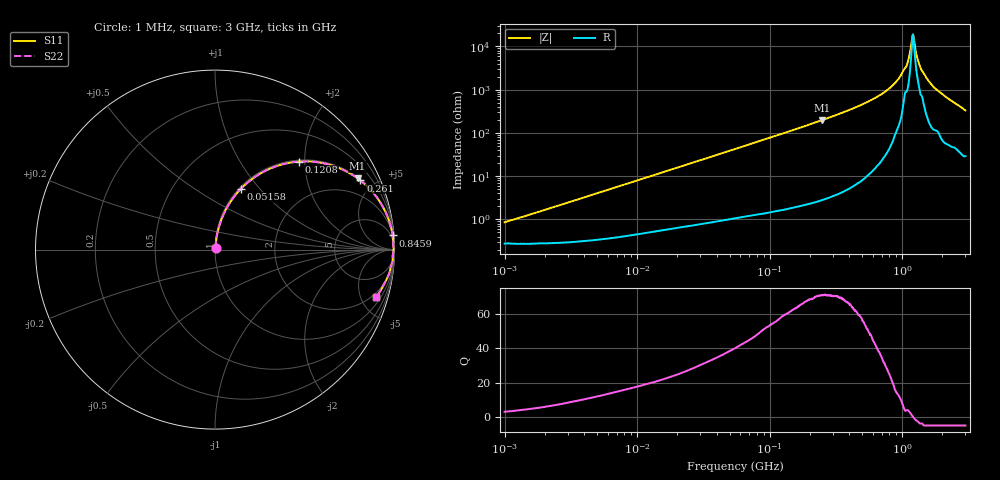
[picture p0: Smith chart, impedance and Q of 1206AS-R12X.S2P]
!s-Parameter Generated by FASTRON Sdn. Bhd.
!FASTRON P/N : 1206AS-R12X
!Keysight Technologies: E4991B_MY54100416_A.01.15
!Date: Wed Nov 15 11:00:45 2023
!Version  :Rev00  Wed Nov 15 11:00:45 2023
!Data & Calibration Information:
!Freq  S11  S21  S12  S22
!PortZ  Port1:50+j0  Port2:50+j0
!When reading reference impedance value at option line is always used.
! Remarks : This data is being provided solely for informational purposes.
# Hz S dB R 50
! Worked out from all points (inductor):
!   1601 points, 1 MHz to 3 GHz, reference 50 ohm
!   read as one part in series: L = 130 nH near 1.041 MHz
!   highest Q = 71 at 249.5 MHz (marker M1), where L = 127 nH
!   self-resonance near 1.207 GHz
!   S11 on the Smith chart (normalised r, x): 1 MHz: 1.01, +0.02; 51.58 MHz: 1.02, +0.80; 120.8 MHz: 1.03, +1.87; 261 MHz: 1.06, +4.17; 845.9 MHz: 2, +25; 3 GHz: 1.58, -6.61
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1000000  -41.33 70.8  -0.02 -0.5  -0.02 -0.5  -41.33 70.8
3804036  -30.23 82.5  -0.03 -1.8  -0.03 -1.8  -30.23 82.5
1.447069e7  -18.94 80.8  -0.10 -6.5  -0.10 -6.5  -18.94 80.8
5.15801e7  -8.69 67.0  -0.72 -21.6  -0.72 -21.6  -8.69 67.0
5.477226e7  -8.25 65.8  -0.80 -22.8  -0.80 -22.8  -8.25 65.8
1.207609e8  -3.39 46.4  -2.80 -42.6  -2.80 -42.6  -3.39 46.4
2.083556e8  -1.43 31.2  -5.72 -58.0  -5.72 -58.0  -1.43 31.2
2.494827e8  -1.03 26.6  -6.99 -62.6  -6.99 -62.6  -1.03 26.6
2.609752e8  -0.95 25.5  -7.33 -63.7  -7.33 -63.7  -0.95 25.5
5.128394e8  -0.22 11.9  -13.73 -77.1  -13.73 -77.1  -0.22 11.9
7.925923e8  -0.07 5.4  -20.48 -82.3  -20.48 -82.3  -0.07 5.4
8.458658e8  -0.06 4.5  -22.02 -82.6  -22.02 -82.6  -0.06 4.5
1.070143e9  -0.07 1.6  -30.65 -73.2  -30.65 -73.2  -0.07 1.6
1.113852e9  -0.05 1.1  -33.88 -73.6  -33.88 -73.6  -0.05 1.1
1.176881e9  -0.04 0.4  -42.01 -50.2  -42.01 -50.2  -0.04 0.4
1.206698e9  -0.05 0.0  -45.61 -1.4  -45.61 -1.4  -0.05 0.0
1.237271e9  -0.05 -0.3  -41.89 45.8  -41.89 45.8  -0.05 -0.3
1.300759e9  -0.06 -1.0  -34.65 67.3  -34.65 67.3  -0.06 -1.0
1.360679e9  -0.07 -1.6  -31.00 73.8  -31.00 73.8  -0.07 -1.6
1.604986e9  -0.08 -3.7  -23.66 80.0  -23.66 80.0  -0.08 -3.7
2.092429e9  -0.18 -7.8  -17.26 77.4  -17.26 77.4  -0.18 -7.8
3e9  -0.58 -16.3  -11.00 68.7  -11.00 68.7  -0.58 -16.3
